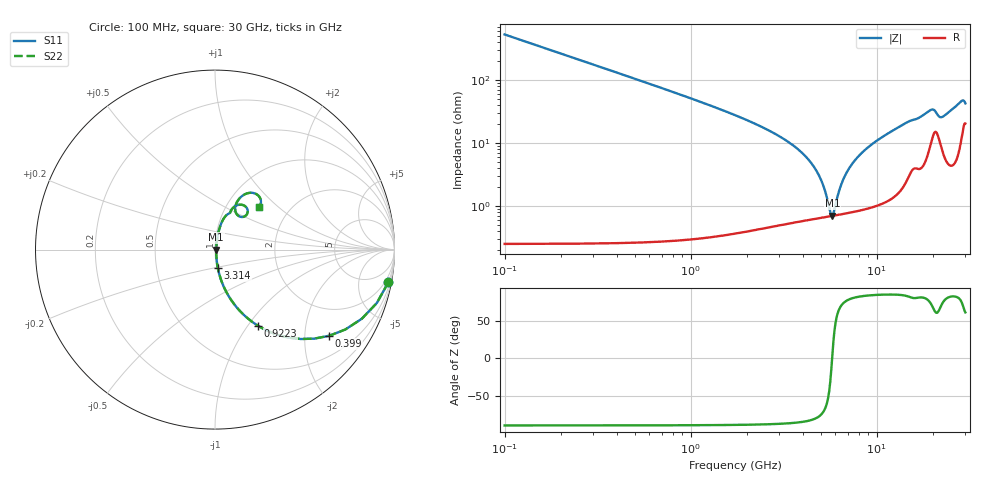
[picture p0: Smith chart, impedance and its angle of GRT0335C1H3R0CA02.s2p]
!Murata Part Number: GRT0335C1H3R0CA02
!These Parameters are Measured in Series Mode Connection
!Data Generated on Jun 19, 2026
!  o--ll--o
!Port1  Port2
!  o------o
!Operation Temp=25[degC], DC Bias Voltage=0[V]
!Freq. Start=100[MHz] Stop=30[GHz] 401[Steps]
# Hz S RI R 50
!Freq.(Hz) S11(Real) S11(Imag) S21(Real) S21(Imag) S12(Real) S12(Imag) S22(Real) S22(Imag)
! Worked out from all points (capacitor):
!   401 points, 100 MHz to 30 GHz, reference 50 ohm
!   read as one part in series: C = 3 pF near 249.5 MHz
!   lowest |Z| = 697 mohm at 5.781 GHz (marker M1)
!   series resonance near 5.764 GHz, so ESL is about 250 pH
!   S11 on the Smith chart (normalised r, x): 100 MHz: 1, -11; 399 MHz: 1.01, -2.65; 922.2 MHz: 1.01, -1.12; 3.314 GHz: 1.01, -0.21; 30 GHz: 1.41, +0.75
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1e8  0.9656 -0.1821  0.0344 0.1821  0.0344 0.1821  0.9656 -0.1821
3.99e8  0.6361 -0.4802  0.3639 0.4802  0.3639 0.4802  0.6361 -0.4802
6.2325e8  0.4144 -0.491  0.5856 0.491  0.5856 0.491  0.4144 -0.491
9.2225e8  0.2397 -0.4243  0.7603 0.4243  0.7603 0.4243  0.2397 -0.4243
1.296e9  0.1327 -0.3351  0.8673 0.3351  0.8673 0.3351  0.1327 -0.3351
1.7445e9  0.0733 -0.254  0.9267 0.254  0.9267 0.254  0.0733 -0.254
3.31425e9  0.0162 -0.104  0.9838 0.104  0.9838 0.104  0.0162 -0.104
4.4355e9  0.00833 -0.0476  0.9917 0.0476  0.9917 0.0476  0.00833 -0.0476
5.10825e9  0.00696 -0.0218  0.993 0.0218  0.993 0.0218  0.00696 -0.0218
5.6315e9  0.00683 -0.00419  0.9932 0.00419  0.9932 0.00419  0.00683 -0.00419
5.781e9  0.00691 0.000535  0.9931 -0.000535  0.9931 -0.000535  0.00691 0.000535
5.9305e9  0.00702 0.00514  0.993 -0.00514  0.993 -0.00514  0.00702 0.00514
6.5285e9  0.00787 0.0225  0.9921 -0.0225  0.9921 -0.0225  0.00787 0.0225
7.20125e9  0.00943 0.0405  0.9906 -0.0405  0.9906 -0.0405  0.00943 0.0405
8.39725e9  0.0135 0.0695  0.9865 -0.0695  0.9865 -0.0695  0.0135 0.0695
1.01165e10  0.0218 0.1071  0.9782 -0.1071  0.9782 -0.1071  0.0218 0.1071
1.505e10  0.073 0.1988  0.927 -0.1988  0.927 -0.1988  0.073 0.1988
2.005825e10  0.1778 0.2304  0.8222 -0.2304  0.8222 -0.2304  0.1778 0.2304
2.200175e10  0.129 0.1891  0.871 -0.1891  0.871 -0.1891  0.129 0.1891
2.50665e10  0.1273 0.2733  0.8727 -0.2733  0.8727 -0.2733  0.1273 0.2733
2.8505e10  0.2261 0.3113  0.7739 -0.3113  0.7739 -0.3113  0.2261 0.3113
3e10  0.2424 0.2347  0.7576 -0.2347  0.7576 -0.2347  0.2424 0.2347
